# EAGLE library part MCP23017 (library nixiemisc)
http://ww1.microchip.com/downloads/en/DeviceDoc/21952a.pdf Source: http://ww1.microchip.com/downloads/en/DeviceDoc/21952a.pdf
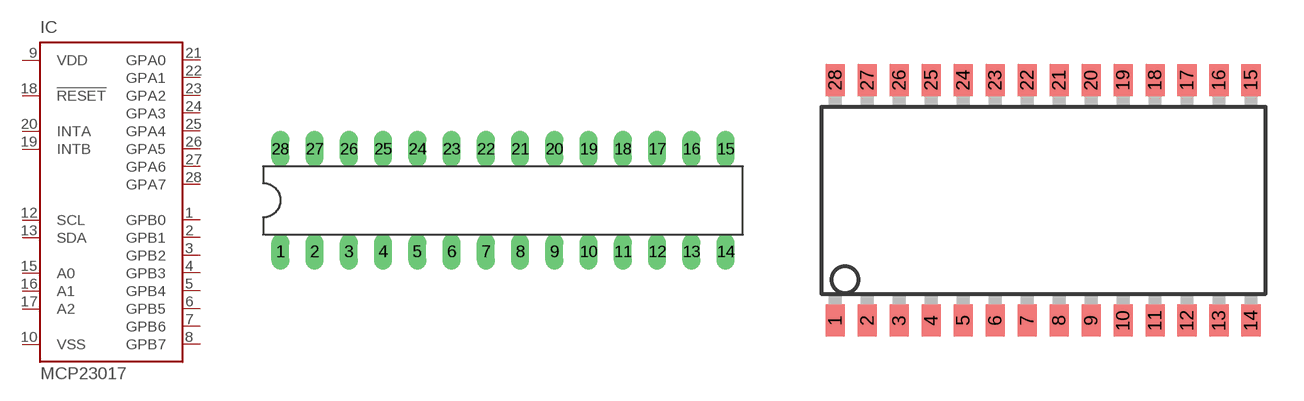
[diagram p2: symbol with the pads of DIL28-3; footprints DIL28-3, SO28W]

Designator prefix IC

## MCP23017SP  [DIL28-3]
1  GPB0
2  GPB1
3  GPB2
4  GPB3
5  GPB4
6  GPB5
7  GPB6
8  GPB7
9  VDD  pwr
10  VSS  pwr
12  SCL  in
13  SDA
15  A0  in
16  A1  in
17  A2  in
18  !RESET  in
19  INTB  out
20  INTA  out
21  GPA0
22  GPA1
23  GPA2
24  GPA3
25  GPA4
26  GPA5
27  GPA6
28  GPA7

## MCP23017SO  [SO28W]
Pads as for DIL28-3

## MCP23017SS  [SSOP28]
Pads as for DIL28-3

## MCP23017ML  [QFN28-ML_6X6MM]
1  GPB4
2  GPB5
3  GPB6
4  GPB7
5  VDD  pwr
6  VSS  pwr
8  SCL  in
9  SDA
11  A0  in
12  A1  in
13  A2  in
14  !RESET  in
15  INTB  out
16  INTA  out
17  GPA0
18  GPA1
19  GPA2
20  GPA3
21  GPA4
22  GPA5
23  GPA6
24  GPA7
25  GPB0
26  GPB1
27  GPB2
28  GPB3

## MCP23017SP2  [DIL28-3-ROUND]
Pads as for DIL28-3

## Footprint DIL28-3 (pad centres in mm)
Dual In Line package type P
drill 0.813 long: 1 -16.51,-3.81; 2 -13.97,-3.81; 3 -11.43,-3.81; 4 -8.89,-3.81; 5 -6.35,-3.81; 6 -3.81,-3.81; 7 -1.27,-3.81; 8 1.27,-3.81; 9 3.81,-3.81; 10 6.35,-3.81; 11 8.89,-3.81; 12 11.43,-3.81; 13 13.97,-3.81; 14 16.51,-3.81; 15 16.51,3.81; 16 13.97,3.81; 17 11.43,3.81; 18 8.89,3.81; 19 6.35,3.81; 20 3.81,3.81; 21 1.27,3.81; 22 -1.27,3.81; 23 -3.81,3.81; 24 -6.35,3.81; 25 -8.89,3.81; 26 -11.43,3.81; 27 -13.97,3.81; 28 -16.51,3.81

## Footprint SO28W (pad centres in mm)
28-Lead Plastic Small Outline (SO) Wide, 300 mil Body (SOIC) Source: http://ww1.microchip.com/downloads/en/devicedoc/39632c.pdf
smd 0.762 x 1.27: 1 -7.62,-4.78; 2 -6.35,-4.78; 3 -5.08,-4.78; 4 -3.81,-4.78; 5 -2.54,-4.78; 6 -1.27,-4.78; 7 0,-4.78; 8 1.27,-4.78; 9 2.54,-4.78; 10 3.81,-4.78; 11 5.08,-4.78; 12 6.35,-4.78; 13 7.62,-4.78; 14 8.89,-4.78; 15 8.89,4.78; 16 7.62,4.78; 17 6.35,4.78; 18 5.08,4.78; 19 3.81,4.78; 20 2.54,4.78; 21 1.27,4.78; 22 0,4.78; 23 -1.27,4.78; 24 -2.54,4.78; 25 -3.81,4.78; 26 -5.08,4.78; 27 -6.35,4.78; 28 -7.62,4.78

## Footprint SSOP28 (pad centres in mm)
Shrink Small Outline Package package type SS
smd 0.4 x 1.5: 1 -4.225,-3.625; 2 -3.575,-3.625; 3 -2.925,-3.625; 4 -2.275,-3.625; 5 -1.625,-3.625; 6 -0.975,-3.625; 7 -0.325,-3.625; 8 0.325,-3.625; 9 0.975,-3.625; 10 1.625,-3.625; 11 2.275,-3.625; 12 2.925,-3.625; 13 3.575,-3.625; 14 4.225,-3.625; 15 4.225,3.625; 16 3.575,3.625; 17 2.925,3.625; 18 2.275,3.625; 19 1.625,3.625; 20 0.975,3.625; 21 0.325,3.625; 22 -0.325,3.625; 23 -0.975,3.625; 24 -1.625,3.625; 25 -2.275,3.625; 26 -2.925,3.625; 27 -3.575,3.625; 28 -4.225,3.625

## Footprint QFN28-ML_6X6MM (pad centres in mm)
QFN28-ML_6X6MM Source: http://www.microchip.com .. 39637a.pdf
smd 1.1 x 0.35: 1 -2.9,1.95; 2 -2.9,1.3; 3 -2.9,0.65; 4 -2.9,0; 5 -2.9,-0.65; 6 -2.9,-1.3; 7 -2.9,-1.95; 15 2.9,-1.95; 16 2.9,-1.3; 17 2.9,-0.65; 18 2.9,0; 19 2.9,0.65; 20 2.9,1.3; 21 2.9,1.95
smd 0.35 x 1.1: 8 -1.95,-2.9; 9 -1.3,-2.9; 10 -0.65,-2.9; 11 0,-2.9; 12 0.65,-2.9; 13 1.3,-2.9; 14 1.95,-2.9; 22 1.95,2.9; 23 1.3,2.9; 24 0.65,2.9; 25 0,2.9; 26 -0.65,2.9; 27 -1.3,2.9; 28 -1.95,2.9
smd 3.7 x 3.7: EXP 0,0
